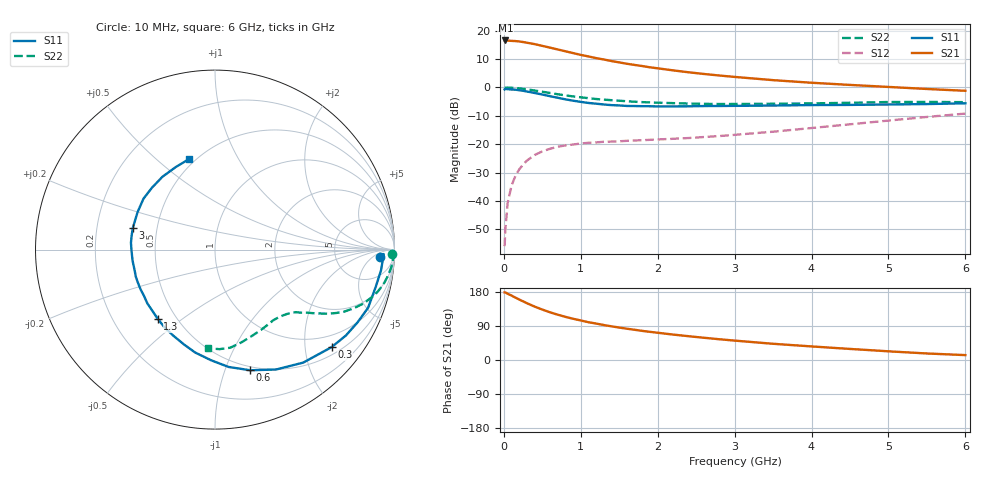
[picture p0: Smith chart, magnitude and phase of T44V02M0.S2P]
! Infineon Technologies  Discrete & RF Semiconductors
! BFR182T
! Si NPN RF Bipolar Junction Transistor in SC75
! VCE = 4 V  IC = 2 mA
! Common Emitter S-Parameters:  October  1999
# GHz  S  MA  R  50
!  f  S11  S21  S12  S22
! GHz  MAG  ANG  MAG  ANG  MAG  ANG  MAG  ANG
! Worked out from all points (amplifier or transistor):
!   36 points, 10 MHz to 6 GHz, reference 50 ohm
!   highest |S21| = 16.5 dB at 20 MHz (marker M1)
!   |S21| within 3 dB of that: start of sweep to 673.2 MHz
!   unconditionally stable (mu >= 1): 2.011 GHz to 4.341 GHz
!   at 250 MHz: K = 0.14, MSG = 21.6 dB, |S12| = -27.2 dB
!   at 1.4 GHz: K = 0.77, MSG = 14.2 dB, |S12| = -19.1 dB
!   at 6 GHz: K = 0.82, MSG = 4.0 dB, |S12| = -9.2 dB
!   lowest NFmin = 1.10 dB at 450 MHz
!   S11 on the Smith chart (normalised r, x): 10 MHz: 19, -10; 300 MHz: 0.68, -2.60; 600 MHz: 0.46, -1.23; 1.3 GHz: 0.40, -0.41; 3 GHz: 0.36, +0.11; 6 GHz: 0.46, +0.65
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0.01  0.9214 -2.5  6.652 178.3  0.0016 76.7  0.9889 -1.3
0.02  0.9404 -1.5  6.717 178.2  0.0032 94.5  0.9873 -1.1
0.05  0.9323 -7.1  6.682 174.8  0.0093 89.5  0.9935 -2.9
0.1  0.9189 -13.3  6.602 170.0  0.0187 82.9  0.9871 -5.7
0.2  0.8916 -27.1  6.447 159.6  0.0361 75.6  0.9624 -10.9
0.3  0.847 -39.9  6.127 149.9  0.0514 68.5  0.9267 -15.7
0.4  0.7988 -52.0  5.79 140.9  0.0645 62.5  0.8823 -19.8
0.5  0.7498 -63.0  5.394 133.1  0.0747 57.5  0.8395 -22.9
0.6  0.7004 -73.7  5.02 125.8  0.0831 53.5  0.7979 -25.7
0.7  0.6582 -83.4  4.662 119.6  0.0901 50.3  0.7584 -27.8
0.8  0.617 -92.0  4.334 113.9  0.0951 47.4  0.7249 -29.5
0.9  0.584 -100.9  4.022 108.8  0.0987 45.5  0.6936 -30.9
1.1  0.5327 -115.9  3.511 99.7  0.1059 42.4  0.6462 -33.2
1.3  0.5004 -129.6  3.105 92.3  0.1105 41.0  0.6092 -35.2
1.5  0.4817 -141.4  2.761 85.6  0.1125 40.9  0.5833 -36.9
1.8  0.4673 -157.1  2.378 76.8  0.1178 41.4  0.5509 -39.9
2.2  0.4634 -172.3  1.997 67.1  0.1245 44.2  0.5289 -43.7
3  0.4735 165.2  1.532 51.2  0.1462 51.4  0.5109 -52.9
3.5  0.4792 154.2  1.343 42.8  0.1661 55.3  0.5153 -59.8
4.5  0.4922 135.6  1.107 29.2  0.2241 58.9  0.5367 -73.8
5.5  0.5093 115.4  0.939 17.2  0.3021 57.1  0.5553 -87.5
6  0.5252 105.8  0.872 12.9  0.3459 54.2  0.5502 -93.8
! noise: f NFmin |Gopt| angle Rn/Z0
0.45  1.1  0.42  29  0.36
0.9  1.2  0.4  58  0.3
1.8  1.85  0.32  126  0.22
